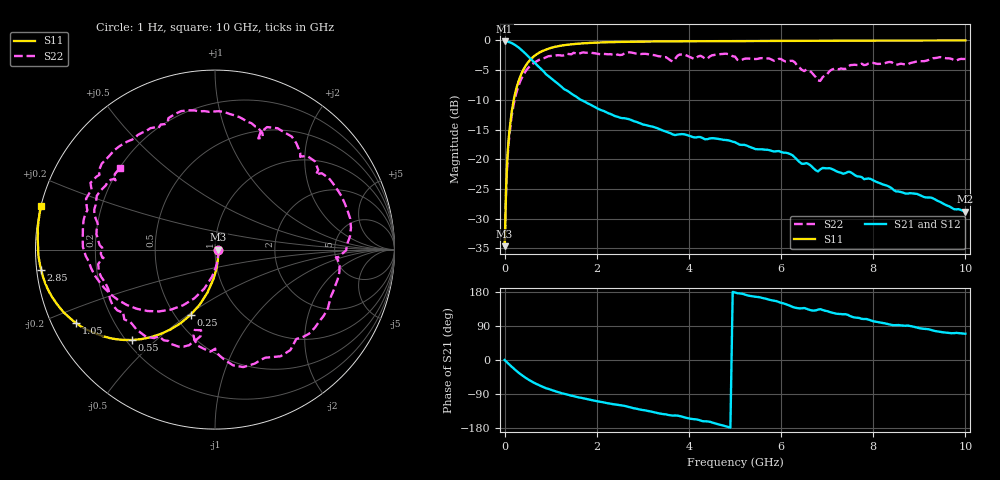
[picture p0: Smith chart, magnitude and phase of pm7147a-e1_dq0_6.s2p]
# GHz S DB R 50
! S-Parameters data
! Freq  dbS11  angS11  dbS21  angS21  dbS12  angS12  dbS22  angS22
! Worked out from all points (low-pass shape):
!   279 points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, 1 Hz to 10 GHz, reference 50 ohm
!   highest |S21| = -0.16 dB at 19.95 kHz (marker M1); lowest = -28.8 dB at 10 GHz (marker M2)
!   |S21| within 3 dB of the highest: start of sweep to 574.5 MHz
!   lowest |S11| = -34.6 dB at 19.95 kHz (marker M3), VSWR 1.04, Z = 51.9 - j0.00344 ohm
!   |S11| at or under -10 dB: start of sweep to 198.3 MHz
!   |S22| runs from -34.6 to -2.0 dB; largest |S21 - S12| = 0
!   S11 on the Smith chart (normalised r, x): 1 Hz: 1.04, -0.00; 250 MHz: 0.60, -0.51; 550 MHz: 0.22, -0.42; 1.05 GHz: 0.07, -0.25; 2.85 GHz: 0.01, -0.06; 10 GHz: 0.00, +0.12
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1e-09  -34.62 -0.0  -0.16 -0.0  -0.16 -0.0  -34.62 -0.0
1.99526e-05  -34.62 -0.1  -0.16 -0.0  -0.16 -0.0  -34.62 -0.1
0.03981072  -23.20 -78.0  -0.19 -4.7  -0.19 -4.7  -23.82 -78.4
0.07943282  -17.50 -89.8  -0.24 -9.3  -0.24 -9.3  -18.15 -92.2
0.25  -8.22 -110.5  -0.89 -28.0  -0.89 -28.0  -8.95 -119.8
0.55  -3.31 -132.5  -2.97 -54.2  -2.97 -54.2  -4.33 -152.4
1.05  -1.17 -152.0  -6.63 -80.5  -6.63 -80.5  -2.59 172.8
1.7  -0.49 -163.7  -10.16 -100.7  -10.16 -100.7  -2.02 142.8
2.85  -0.22 -173.4  -13.68 -128.1  -13.68 -128.1  -2.21 96.7
3.35  -0.17 -175.9  -14.89 -140.9  -14.89 -140.9  -2.68 75.9
4.45  -0.12 179.7  -16.50 -162.9  -16.50 -162.9  -2.72 35.6
4.8  -0.12 178.6  -16.75 -174.6  -16.75 -174.6  -2.24 12.9
5.05  -0.11 177.9  -17.34 176.3  -17.34 176.3  -3.26 -3.5
5.55  -0.09 176.4  -18.32 165.2  -18.32 165.2  -2.99 -27.4
6  -0.09 175.2  -18.76 150.8  -18.76 150.8  -3.13 -58.5
6.25  -0.08 174.6  -19.33 140.1  -19.33 140.1  -3.44 -76.4
6.7  -0.05 173.4  -21.49 130.4  -21.49 130.4  -5.72 -102.7
6.9  -0.05 172.9  -21.46 132.0  -21.46 132.0  -6.22 -99.5
7.5  -0.04 171.4  -22.14 115.9  -22.14 115.9  -4.16 -128.3
8.35  -0.02 169.4  -24.63 94.0  -24.63 94.0  -3.63 -169.3
9.3  -0.01 167.3  -26.58 77.6  -26.58 77.6  -2.99 161.6
10  -0.01 165.8  -28.79 69.2  -28.79 69.2  -3.12 139.4
